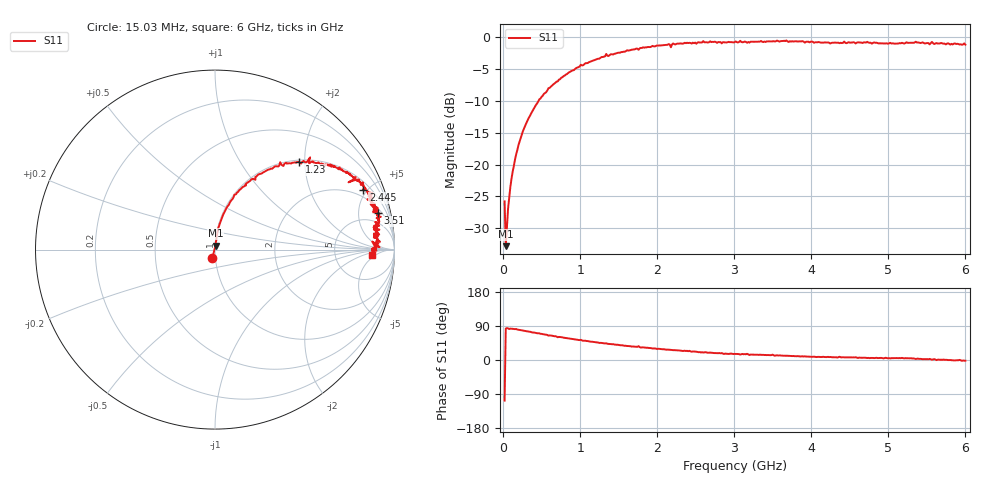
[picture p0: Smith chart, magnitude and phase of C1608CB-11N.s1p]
!	Network	Analyzer	HP8753E.07.74:	Oct	30	2002	Serial	No.	JP38451487
!	Hewlett-Packard
!	28	Aug	2009	7:53:39
!	Frequency	S11
#	HZ	S	RI	R	50
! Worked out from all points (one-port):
!   400 points, 15.03 MHz to 6 GHz, reference 50 ohm
!   lowest |S11| = -32.8 dB at 30.03 MHz (marker M1), VSWR 1.05, Z = 50.2 + j2.28 ohm
!   |S11| at or under -10 dB: start of sweep to 456 MHz
!   S11 on the Smith chart (normalised r, x): 15.03 MHz: 0.97, -0.10; 1.23 GHz: 1.04, +1.88; 2.445 GHz: 1.47, +4.74; 3.51 GHz: 2.76, +8.17; 6 GHz: 14, -3
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1.502992e7  -0.0152 -0.0491
3.002985e7  0.0028 0.0227
6.00297e7  0.00525 0.0448
1.050295e8  0.0103 0.077
1.650292e8  0.0171 0.119
2.550287e8  0.0397 0.18
4.650277e8  0.108 0.306
7.650262e8  0.243 0.419
1.005025e9  0.363 0.487
1.230024e9  0.47 0.488
1.515022e9  0.587 0.475
1.725021e9  0.668 0.464
1.755021e9  0.64 0.474
1.785021e9  0.691 0.447
1.93502e9  0.737 0.431
2.145019e9  0.784 0.404
2.175019e9  0.744 0.375
2.205019e9  0.802 0.39
2.265019e9  0.804 0.384
2.445018e9  0.827 0.332
2.595017e9  0.876 0.315
2.835016e9  0.849 0.28
3.015015e9  0.889 0.257
3.510012e9  0.907 0.202
3.765011e9  0.908 0.17
4.515007e9  0.9 0.113
5.265004e9  0.9 0.0692
6e9  0.872 -0.0278
